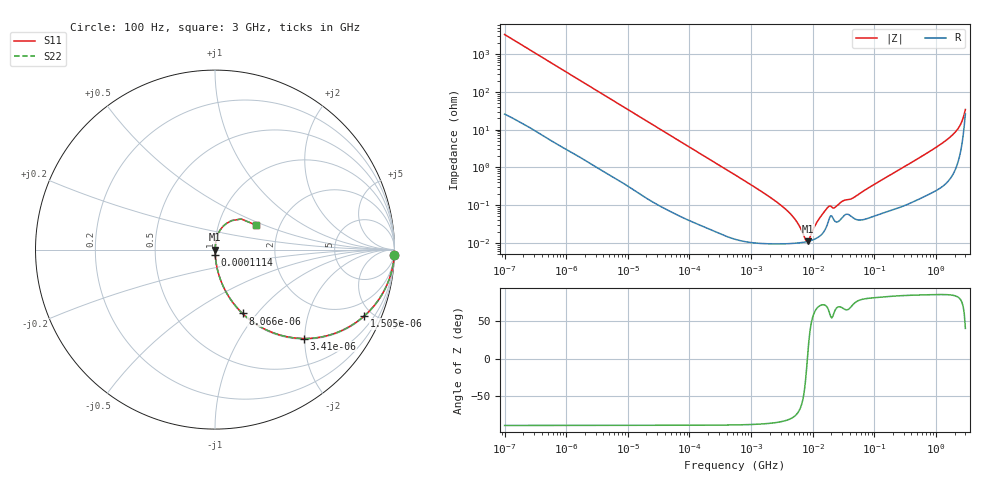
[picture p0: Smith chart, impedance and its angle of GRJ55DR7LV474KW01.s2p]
!Murata Part Number: GRJ55DR7LV474KW01
!These Parameters are Measured in Series Mode Connection
!Data Generated on Jun 19, 2026
!  o--ll--o
!Port1  Port2
!  o------o
!Operation Temp=25[degC], DC Bias Voltage=0[V]
!Freq. Start=100[Hz] Stop=3[GHz] 401[Steps]
# Hz S RI R 50
!Freq.(Hz) S11(Real) S11(Imag) S21(Real) S21(Imag) S12(Real) S12(Imag) S22(Real) S22(Imag)
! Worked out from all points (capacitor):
!   401 points, 100 Hz to 3 GHz, reference 50 ohm
!   read as one part in series: C = 479 nF near 109 Hz
!   lowest |Z| = 10.9 mohm at 8.245 MHz (marker M1)
!   series resonance near 8.187 MHz, so ESL is about 790 pH
!   S11 on the Smith chart (normalised r, x): 100 Hz: 2, -66; 1.505 kHz: 1.04, -4.47; 3.41 kHz: 1.02, -1.98; 8.066 kHz: 1.01, -0.84; 111.4 kHz: 1.00, -0.06; 3 GHz: 1.52, +0.44
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100  0.9989 -0.0301  0.00114 0.0301  0.00114 0.0301  0.9989 -0.0301
451  0.981 -0.1321  0.019 0.1321  0.019 0.1321  0.981 -0.1321
1505  0.8312 -0.37  0.1688 0.37  0.1688 0.37  0.8312 -0.37
1788  0.7783 -0.4108  0.2217 0.4108  0.2217 0.4108  0.7783 -0.4108
3410  0.4962 -0.4954  0.5038 0.4954  0.5038 0.4954  0.4962 -0.4954
8066  0.1534 -0.3557  0.8466 0.3557  0.8466 0.3557  0.1534 -0.3557
31977  0.0123 -0.1058  0.9877 0.1058  0.9877 0.1058  0.0123 -0.1058
111411  0.00132 -0.0309  0.9987 0.0309  0.9987 0.0309  0.00132 -0.0309
547723  0.000165 -0.00633  0.9998 0.00633  0.9998 0.00633  0.000165 -0.00633
3639519  9.52e-05 -0.000772  0.9999 0.000772  0.9999 0.000772  9.52e-05 -0.000772
5361412  9.83e-05 -0.000375  0.9999 0.000375  0.9999 0.000375  9.83e-05 -0.000375
7565221  0.000106 -6.84e-05  0.9999 6.84e-05  0.9999 6.84e-05  0.000106 -6.84e-05
8245314  0.000109 6.3e-06  0.9999 -6.3e-06  0.9999 -6.3e-06  0.000109 6.3e-06
9794414  0.000118 0.000159  0.9999 -0.000159  0.9999 -0.000159  0.000118 0.000159
1.268047e7  0.000146 0.000408  0.9999 -0.000408  0.9999 -0.000408  0.000146 0.000408
1.789277e7  0.000367 0.000825  0.9996 -0.000825  0.9996 -0.000825  0.000367 0.000825
2.316512e7  0.000368 0.000798  0.9996 -0.000798  0.9996 -0.000798  0.000368 0.000798
4.418008e7  0.000476 0.00144  0.9995 -0.00144  0.9995 -0.00144  0.000476 0.00144
1.751444e8  0.000736 0.00603  0.9993 -0.00603  0.9993 -0.00603  0.000736 0.00603
1.573002e9  0.00747 0.0564  0.9925 -0.0564  0.9925 -0.0564  0.00747 0.0564
2.219584e9  0.0215 0.0963  0.9785 -0.0963  0.9785 -0.0963  0.0215 0.0963
3e9  0.2297 0.1358  0.7703 -0.1358  0.7703 -0.1358  0.2297 0.1358
